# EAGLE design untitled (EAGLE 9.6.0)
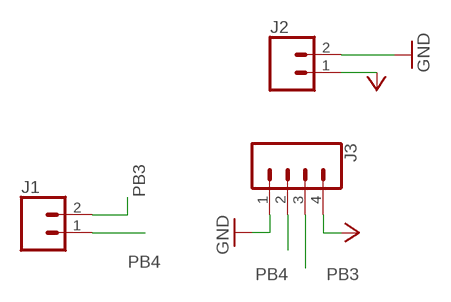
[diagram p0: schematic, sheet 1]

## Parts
J1  CONN_02  [1X02]
J2  CONN_02  [1X02]
J3  CONN_04POLAR  [MOLEX-1X4]

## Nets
GND: J2.2 J3.1
PB3: J1.2 J3.3
PB4: J1.1 J3.2
VCC: J2.1 J3.4

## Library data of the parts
J1 J2 = SparkFun-Connectors:CONN_02: Multi connection point. Often used as Generic Header-pin footprint for 0.1 inch spaced/style header connections
J3 = SparkFun-Connectors:CONN_04: Multi connection point. Often used as Generic Header-pin footprint for 0.1 inch spaced/style header connections On any of the 0.1 inch spaced packages, you can populate with these: Break Away Headers - Straight (PRT-00116) Break Away Male Headers - Right Angle (PRT-00553) Female Headers (PRT-00115)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; PROD_ID: CONN-08186; SF_ID: PRT-08231

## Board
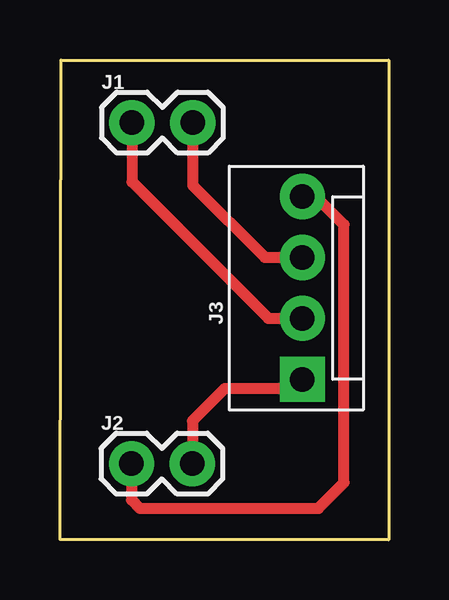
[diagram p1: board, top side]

Size 13.72 x 19.99 mm. Coordinates in mm from the lower left corner, seen from the top.
Outline: 0.05,19.99 13.72,19.98 13.71,0 0,0 0.05,19.99
Copper layers (1*16): Top 0.035mm / dielectric 1.5mm / Bottom 0.035mm
Design rules "default *": minimum track width 18mil, minimum drill 0.35mm, track to track 16mil, track to pad 16mil, pad to pad 16mil, via to via 6mil, smd to smd 16mil, copper to edge 40mil, drill to drill 6mil, minimum pad ring 10mil, minimum via ring 8mil, stop-mask expansion 4mil, vias tented up to drill 0mil, thermal gap 10mil

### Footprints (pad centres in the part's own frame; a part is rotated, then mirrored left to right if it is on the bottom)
1X02 = drill 1.016 pad 1.88: 1 0,0; 2 2.54,0
MOLEX-1X4 = drill 1.016 pad 1.88 square: 1 0,0 | drill 1.016 pad 1.88: 2 2.54,0; 3 5.08,0; 4 7.62,0

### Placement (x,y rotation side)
J1  3,17.38 0 top
J2  2.98,3.17 0 top
J3  10.11,6.68 90 top

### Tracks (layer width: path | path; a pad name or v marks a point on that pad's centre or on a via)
GND
  Top 0.457: J3.1 9.73,6.3 6.87,6.3 5.52,4.96 J2.2
PB3
  Top 0.457: J1.2 5.54,14.77 8.55,11.76 J3.3
PB4
  Top 0.457: J1.1 3,14.91 8.69,9.22 J3.2
VCC
  Top 0.457: J2.1 2.98,1.66 3.33,1.31 10.78,1.31 11.85,2.38 11.85,13.13 10.68,14.3 J3.4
